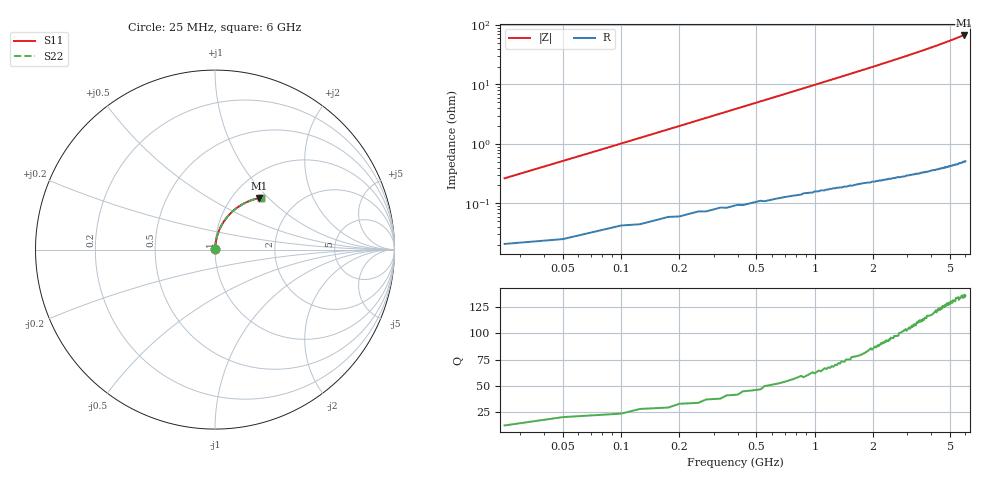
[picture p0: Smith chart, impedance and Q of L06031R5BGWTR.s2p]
!	AVX Thin Film Operation
!	Date:	March	2003
!	Description: Accu-L® Series Thin Film SMD RF Inductors
!	Part Number: L06031R5BGWTR
!	25MHz-6GHz
!	Serial	Measurements
#	mhz	S	db	R	50
!	S11	S11	S21	S21	S12	S12	S22	S22
!	dB	Phase	dB	Phase	dB	Phase	dB	Phase
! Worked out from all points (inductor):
!   240 points, 25 MHz to 6 GHz, reference 50 ohm
!   read as 1/Y11, port 2 shorted: L = 1.62 nH near 50 MHz
!   highest Q = 135 at 5.9 GHz (marker M1), where L = 1.82 nH
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25  -54.09 84.4  -0.00 -0.2  -0.00 -0.2  -54.09 84.4
50  -48.35 85.5  -0.00 -0.4  -0.00 -0.4  -48.35 85.5
75  -44.96 85.9  -0.00 -0.6  -0.00 -0.6  -44.96 85.9
100  -42.55 86.1  -0.00 -0.7  -0.00 -0.7  -42.55 86.1
125  -40.67 86.2  -0.00 -0.9  -0.00 -0.9  -40.67 86.2
175  -37.83 86.2  -0.01 -1.3  -0.01 -1.3  -37.83 86.2
225  -35.70 86.1  -0.01 -1.6  -0.01 -1.6  -35.70 86.1
275  -33.99 85.9  -0.01 -2.0  -0.01 -2.0  -33.99 85.9
325  -32.57 85.7  -0.01 -2.3  -0.01 -2.3  -32.57 85.7
400  -30.80 85.3  -0.01 -2.9  -0.01 -2.9  -30.80 85.3
575  -27.71 84.3  -0.02 -4.1  -0.02 -4.1  -27.71 84.3
775  -25.16 83.1  -0.03 -5.5  -0.03 -5.5  -25.16 83.1
1025  -22.78 81.5  -0.04 -7.3  -0.04 -7.3  -22.78 81.5
1225  -21.26 80.2  -0.05 -8.7  -0.05 -8.7  -21.26 80.2
1475  -19.68 78.5  -0.06 -10.5  -0.06 -10.5  -19.68 78.5
2025  -17.00 74.8  -0.11 -14.3  -0.11 -14.3  -17.00 74.8
2500  -15.24 71.6  -0.15 -17.6  -0.15 -17.6  -15.24 71.6
3025  -13.66 68.1  -0.22 -21.3  -0.22 -21.3  -13.66 68.1
4025  -11.35 61.5  -0.36 -28.1  -0.36 -28.1  -11.35 61.5
5025  -9.63 54.9  -0.54 -34.7  -0.54 -34.7  -9.63 54.9
5900  -8.43 49.3  -0.71 -40.4  -0.71 -40.4  -8.43 49.3
6000  -8.31 48.7  -0.73 -41.1  -0.73 -41.1  -8.31 48.7
